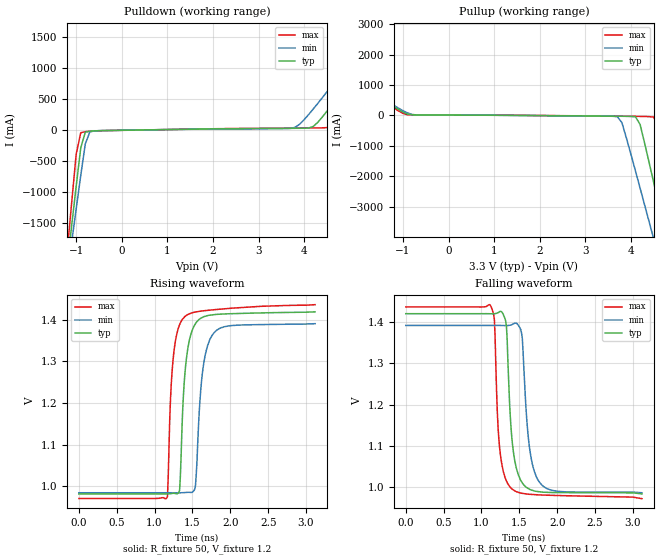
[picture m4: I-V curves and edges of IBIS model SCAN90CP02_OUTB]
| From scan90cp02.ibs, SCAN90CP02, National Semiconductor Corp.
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[Model]   SCAN90CP02_OUTB
Model_type Output
Polarity Inverting
Vref=1.2
Vmeas=1.2
Rref=50   | 100 Ohms Across Outputs OUT+ and OUT-
Cref=1p
C_comp   8pF   8pF   8pF
[Temperature Range] 25   85   -40
[Voltage Range]   3.3   3.0   3.6
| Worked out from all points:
|   slope of the pulldown table from 0 to 0.495 V, typ, clamps not added: 84.1 ohm
|   slope of the pullup table from 0 to 0.495 V, typ, clamps not added: 210 ohm
|   falling waveform, R_fixture 50, V_fixture 1.2: 20-80 % time 89.6ps typ, 105ps min, 77.8ps max; typ from 1.42 V to 0.983 V
|   rising waveform, R_fixture 50, V_fixture 1.2: 20-80 % time 89.8ps typ, 101ps min, 83.9ps max; typ from 0.981 V to 1.42 V
[Pulldown]
|V(pulldown)   I(typ)   I(min)   I(max)
-3.6V     -17.92A    -15.75A    -21.54A
-1.2V     -2.195A    -2.367A    -1.985A
-1.1V     -1.548A    -1.817A    -1.18A
-1V       -908.9mA   -1.271A    -391.3mA
-900mV    -289.9mA   -736mA     -45.84mA
-700mV    -22.24mA   -32.94mA   -22.09mA
3.7V      24.24mA    23.61mA    28.16mA
4.5V      299.2mA    610.9mA    36.3mA
5.6V      1.408A     1.668A     1.121A
5.8V      1.614A     1.863A     1.342A
6.1V      1.925A     2.156A     1.675A
7.2V      3.072A     3.237A     2.903A
[Pullup]
|V(pullup)   I(typ)   I(min)   I(max)
-3.6V     2.74A      2.632A     2.88A
-900mV    43.34mA    80.56mA    22.72mA
3.7V      -26.74mA   -42.08mA   -25.25mA
3.8V      -28.09mA   -232.2mA   -26.59mA
4.1V      -47.53mA   -1.832A    -30.63mA
4.2V      -296.4mA   -2.387A    -32.38mA
4.5V      -2.212A    -4.064A    -54.8mA
4.6V      -2.868A    -4.625A    -397.6mA
4.8V      -4.186A    -5.747A    -1.996A
5V        -5.506A    -6.87A     -3.632A
5.1V      -6.167A    -7.431A    -4.453A
7.2V      -19.97A    -19.17A    -21.64A
[Ramp]
|   typ   min   max
dV/dt_r   320mV/.145ns   310mV/.160ns   330mV/0.120ns
dV/dt_f   320mv/.120ns   310mv/.130ns   330mv/0.100ns
R_load=50
[Falling Waveform]
R_fixture=50
V_fixture=1.2
V_fixture_min=1.18814
V_fixture_max=1.20375
0s        1.421V     1.392V     1.437V
1.12ns    1.421V     1.392V     1.44V
1.17ns    1.421V     1.392V     1.408V
1.23ns    1.425V     1.392V     1.116V
1.32ns    1.403V     1.392V     1.019V
1.41ns    1.103V     1.395V     993.8mV
1.53ns    1.012V     1.374V     984.5mV
1.63ns    994.8mV    1.102V     982mV
1.78ns    987.8mV    1.008V     980.3mV
3.12ns    982.9mV    985.7mV    971.3mV
[Rising Waveform]
R_fixture=50
V_fixture=1.2
V_fixture_min=1.2
V_fixture_max=1.2
0s        981.3mV    984.2mV    970.5mV
1.17ns    981.3mV    984.2mV    974.8mV
1.23ns    982.5mV    984.2mV    1.273V
1.33ns    989.2mV    984.1mV    1.388V
1.37ns    1.178V     984.3mV    1.402V
1.41ns    1.289V     984.8mV    1.409V
1.54ns    1.391V     1.001V     1.419V
1.63ns    1.406V     1.269V     1.421V
1.78ns    1.412V     1.368V     1.424V
3.12ns    1.419V     1.391V     1.436V
